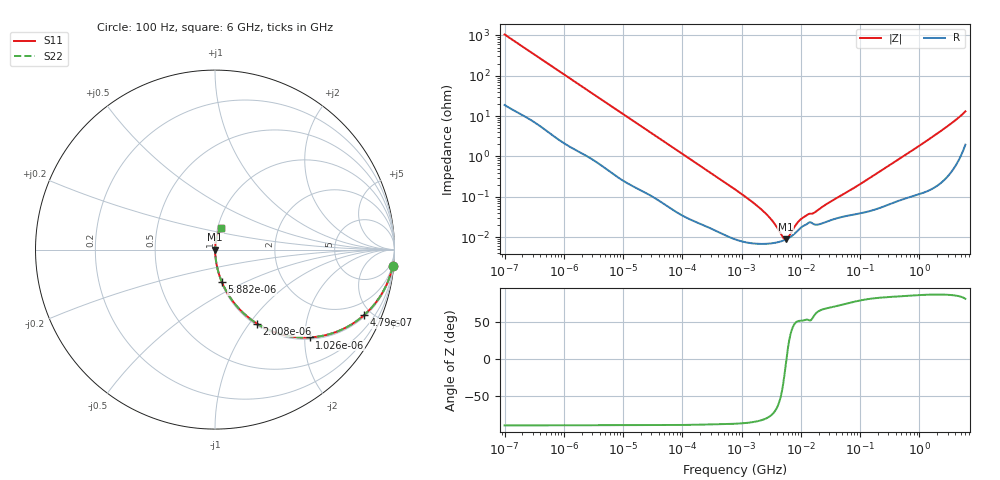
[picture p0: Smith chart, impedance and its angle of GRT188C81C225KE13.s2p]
!Murata Part Number: GRT188C81C225KE13
!These Parameters are Measured in Series Mode Connection
!Data Generated on Jun 19, 2026
!  o--ll--o
!Port1  Port2
!  o------o
!Operation Temp=25[degC], DC Bias Voltage=0[V]
!Freq. Start=100[Hz] Stop=6[GHz] 401[Steps]
# Hz S RI R 50
!Freq.(Hz) S11(Real) S11(Imag) S21(Real) S21(Imag) S12(Real) S12(Imag) S22(Real) S22(Imag)
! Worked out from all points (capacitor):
!   401 points, 100 Hz to 6 GHz, reference 50 ohm
!   read as one part in series: C = 1.5 uF near 109 Hz
!   lowest |Z| = 8.8 mohm at 5.555 MHz (marker M1)
!   series resonance near 5.714 MHz, so ESL is about 520 pH
!   S11 on the Smith chart (normalised r, x): 100 Hz: 1, -21; 479 Hz: 1.09, -4.49; 1.026 kHz: 1.04, -2.12; 2.008 kHz: 1.02, -1.09; 5.882 kHz: 1.01, -0.38; 6 GHz: 1.04, +0.26
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100  0.9894 -0.0937  0.0106 0.0937  0.0106 0.0937  0.9894 -0.0937
245  0.9458 -0.2163  0.0542 0.2163  0.0542 0.2163  0.9458 -0.2163
479  0.8295 -0.3659  0.1705 0.3659  0.1705 0.3659  0.8295 -0.3659
1026  0.5278 -0.4895  0.4722 0.4895  0.4722 0.4895  0.5278 -0.4895
2008  0.2339 -0.4125  0.7661 0.4125  0.7661 0.4125  0.2339 -0.4125
3287  0.1068 -0.2975  0.8932 0.2975  0.8932 0.2975  0.1068 -0.2975
5882  0.0384 -0.1812  0.9616 0.1812  0.9616 0.1812  0.0384 -0.1812
13772  0.0085 -0.0808  0.9915 0.0808  0.9915 0.0808  0.0085 -0.0808
40335  0.00161 -0.0283  0.9984 0.0283  0.9984 0.0283  0.00161 -0.0283
774597  9.09e-05 -0.00153  0.9999 0.00153  0.9999 0.00153  9.09e-05 -0.00153
2372521  6.83e-05 -0.000424  0.9999 0.000424  0.9999 0.000424  6.83e-05 -0.000424
3394479  7.12e-05 -0.000232  0.9999 0.000232  0.9999 0.000232  7.12e-05 -0.000232
4856642  8.06e-05 -6.94e-05  0.9999 6.94e-05  0.9999 6.94e-05  8.06e-05 -6.94e-05
5554849  8.72e-05 -1.19e-05  0.9999 1.19e-05  0.9999 1.19e-05  8.72e-05 -1.19e-05
6353432  9.68e-05 4.52e-05  0.9999 -4.52e-05  0.9999 -4.52e-05  9.68e-05 4.52e-05
8311524  0.000133 0.000157  0.9999 -0.000157  0.9999 -0.000157  0.000133 0.000157
9941735  0.000171 0.000218  0.9998 -0.000218  0.9998 -0.000218  0.000171 0.000218
1.300572e7  0.000217 0.000291  0.9998 -0.000291  0.9998 -0.000291  0.000217 0.000291
1.555665e7  0.000222 0.000312  0.9998 -0.000312  0.9998 -0.000312  0.000222 0.000312
3.124326e8  0.000688 0.006  0.9993 -0.006  0.9993 -0.006  0.000688 0.006
2.048624e9  0.00333 0.0375  0.9967 -0.0375  0.9967 -0.0375  0.00333 0.0375
6e9  0.0348 0.1227  0.9652 -0.1227  0.9652 -0.1227  0.0348 0.1227
